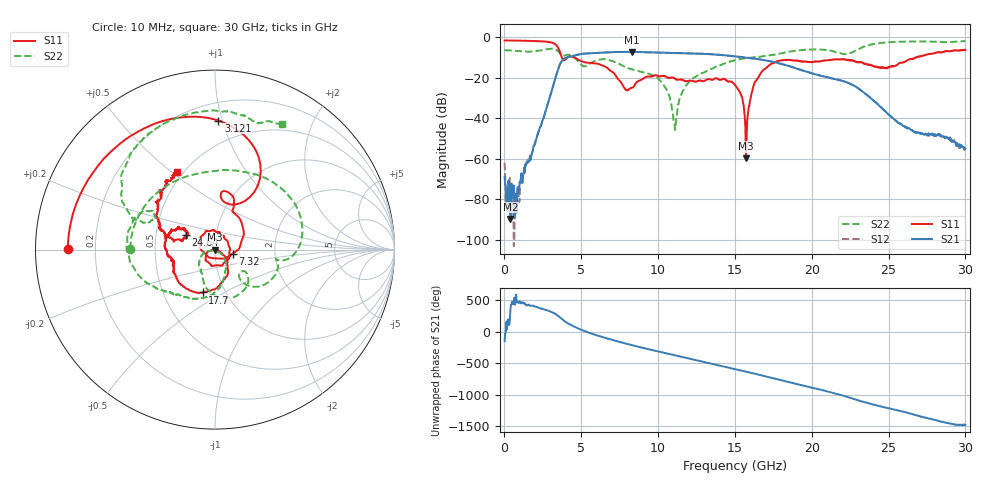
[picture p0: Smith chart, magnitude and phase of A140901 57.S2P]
!  2-Port S-parameters saved by WinCal
! VAR MeasName=S-Parameters (CALIBRATED_DATA) read from VNA (N5244A)
! VAR MeasDate=11/3/2014 9:36:24 AM
! VAR NAME=A140901 57
! VAR FILENAME=A140901 57.S2P
! VAR DATE=11/3/2014 9:36:24 AM
! VAR PHYS_PORTS=1,2
# Hz S RI R 50
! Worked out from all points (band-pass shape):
!   801 points, 10 MHz to 30 GHz, reference 50 ohm
!   highest |S21| = -7.34 dB at 8.295 GHz (marker M1); lowest = -89.6 dB at 384.9 MHz (marker M2)
!   |S21| within 3 dB of the highest: 3.978 GHz to 15.92 GHz (11.94 GHz wide, 120 % of centre)
!   lowest |S11| = -59.7 dB at 15.72 GHz (marker M3), VSWR 1.00, Z = 50 - j0.0977 ohm
!   |S11| at or under -10 dB: 3.726 GHz to 4.115 GHz (389.9 MHz wide, 9.94 % of centre); 4.516 GHz to 26.83 GHz (22.31 GHz wide, 142 % of centre)
!   |S22| runs from -45.7 to -2.0 dB; largest |S21 - S12| = 0.0034
!   S11 on the Smith chart (normalised r, x): 10 MHz: 0.10, +0.00; 3.121 GHz: 0.33, +0.97; 7.32 GHz: 1.22, -0.06; 17.7 GHz: 0.78, -0.40; 24.64 GHz: 0.71, +0.12; 30 GHz: 0.47, +0.52
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1e7  -0.8182 0.00263  -0.000315 -0.000169  0.000351 0.00071  -0.4712 0.00444
3.84875e8  -0.8085 0.1254  3.05e-05 -1.33e-05  0.000125 0.000181  -0.4335 0.1711
8.722125e8  -0.7629 0.2787  -9.46e-05 0.00018  -1.65e-05 0.000142  -0.306 0.3292
3.121462e9  0.0193 0.7191  0.0326 -0.0434  0.0325 -0.0433  0.469 0.2041
3.946188e9  0.0434 0.2722  -0.2855 0.0948  -0.2853 0.0946  0.3463 -0.0641
5.033325e9  0.1017 0.2281  0.3377 0.1779  0.3375 0.1779  0.1345 -0.1503
6.232925e9  0.1494 0.1459  0.1078 -0.3951  0.1078 -0.3942  0.1477 -0.237
7.320062e9  0.098 -0.0234  -0.375 -0.2056  -0.3742 -0.2058  -0.0388 -0.224
8.294738e9  -0.0444 -0.0349  -0.3563 0.2403  -0.3554 0.2396  -0.0709 -0.1438
1.001916e10  -0.0356 0.1033  0.2923 0.2909  0.2914 0.2903  -0.0835 -0.0423
1.11063e10  0.0297 0.089  0.3886 -0.1073  0.3884 -0.1072  -0.000682 -0.00512
1.208098e10  0.0687 0.0487  0.1389 -0.3688  0.1391 -0.3683  0.0559 -0.0606
1.365545e10  0.0455 -0.0807  -0.3439 -0.1413  -0.3439 -0.1406  0.0465 -0.1707
1.5005e10  -0.0514 -0.0393  -0.1954 0.2696  -0.1936 0.2694  -0.0446 -0.2638
1.541736e10  -0.0346 -0.00769  -0.0688 0.3125  -0.0688 0.3119  -0.0897 -0.2744
1.571726e10  -0.000359 -0.000977  0.0264 0.3094  0.0246 0.3078  -0.1233 -0.2756
1.635455e10  0.0664 -0.0476  0.193 0.2148  0.1909 0.2159  -0.1819 -0.262
1.77041e10  -0.0676 -0.2389  0.1956 -0.1278  0.1961 -0.1274  -0.302 -0.2219
2.002832e10  -0.2339 -0.0616  -0.1251 -0.0197  -0.1256 -0.0208  -0.4887 0.0438
2.463929e10  -0.1608 0.0796  -0.00764 -0.0147  -0.00762 -0.0149  -0.4518 0.5634
2.501416e10  -0.1623 0.0652  -0.00906 -0.00811  -0.00912 -0.00816  -0.3859 0.6325
3e10  -0.2093 0.4322  0.00132 -0.00121  0.00109 -0.00109  0.3735 0.7004
